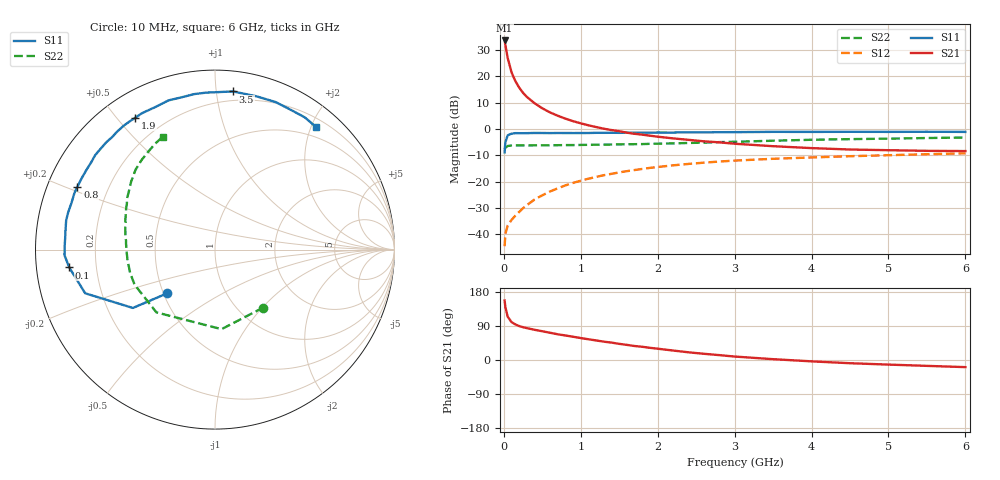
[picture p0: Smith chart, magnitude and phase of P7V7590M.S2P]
! SIEMENS Small Signal Semiconductors
! BFP196
! Si NPN RF Bipolar Junction Transistor in SOT143
! VCE = 0.75 V  IC = 90 mA
! Common Emitter S-Parameters:  May  1996
# GHz  S  MA  R  50
!  f  S11  S21  S12  S22
! GHz  MAG  ANG  MAG  ANG  MAG  ANG  MAG  ANG
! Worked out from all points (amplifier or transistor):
!   36 points, 10 MHz to 6 GHz, reference 50 ohm
!   highest |S21| = 33.7 dB at 10 MHz (marker M1)
!   |S21| within 3 dB of that: start of sweep to 27.9 MHz
!   unconditionally stable (mu >= 1): start of sweep to 14.7 MHz; 171.4 MHz to end of sweep
!   at 250 MHz: K = 1.14, MAG = 19.6 dB, |S12| = -30.0 dB
!   at 1.4 GHz: K = 1.22, MAG = 5.5 dB, |S12| = -17.0 dB
!   at 6 GHz: K = 1.09, MAG = -1.4 dB, |S12| = -9.2 dB
!   S11 on the Smith chart (normalised r, x): 10 MHz: 0.52, -0.29; 100 MHz: 0.10, -0.06; 800 MHz: 0.09, +0.22; 1.9 GHz: 0.10, +0.56; 3.5 GHz: 0.13, +1.11; 6 GHz: 0.33, +2.08
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0.01  0.3616 -137.6  48.19 157.0  0.006 60.8  0.4205 -50.1
0.02  0.5613 -144.6  39.66 139.3  0.0103 54.2  0.4448 -85.3
0.05  0.7631 -161.4  22.38 114.2  0.0148 41.0  0.4784 -133.0
0.1  0.8182 -173.0  11.97 100.0  0.0189 45.4  0.4888 -156.4
0.15  0.8392 -177.9  8.135 93.8  0.0228 50.3  0.4904 -164.8
0.2  0.8376 178.4  6.123 89.5  0.0269 55.9  0.4892 -169.3
0.25  0.8374 175.4  4.874 86.5  0.0316 59.2  0.4913 -172.5
0.3  0.839 173.5  4.078 84.1  0.0361 61.0  0.4908 -174.4
0.4  0.8451 168.9  3.095 79.7  0.0462 63.9  0.4919 -177.4
0.5  0.8439 165.7  2.484 75.9  0.0554 64.7  0.493 -179.6
0.6  0.8409 161.8  2.075 71.9  0.0655 64.9  0.4943 178.6
0.7  0.8442 158.1  1.796 67.9  0.0751 64.3  0.4957 177.1
0.8  0.843 155.4  1.581 64.7  0.0855 63.3  0.4972 175.8
1.1  0.8438 144.9  1.18 54.7  0.1144 59.8  0.5033 171.8
1.4  0.8511 135.4  0.959 45.9  0.1417 55.0  0.5105 168.1
1.9  0.8587 121.1  0.75 32.1  0.1837 46.5  0.5255 162.0
2.2  0.861 112.8  0.667 25.0  0.2054 41.4  0.5356 158.0
3  0.876 93.2  0.528 9.1  0.2525 28.2  0.5751 147.1
3.5  0.8867 83.5  0.474 2.2  0.2734 20.7  0.6021 140.8
4.5  0.8886 67.7  0.41 -8.5  0.306 8.2  0.6454 129.3
5.5  0.8905 55.8  0.387 -15.5  0.3339 -2.6  0.6773 119.6
6  0.885 50.4  0.383 -18.8  0.347 -8.4  0.6931 114.8
